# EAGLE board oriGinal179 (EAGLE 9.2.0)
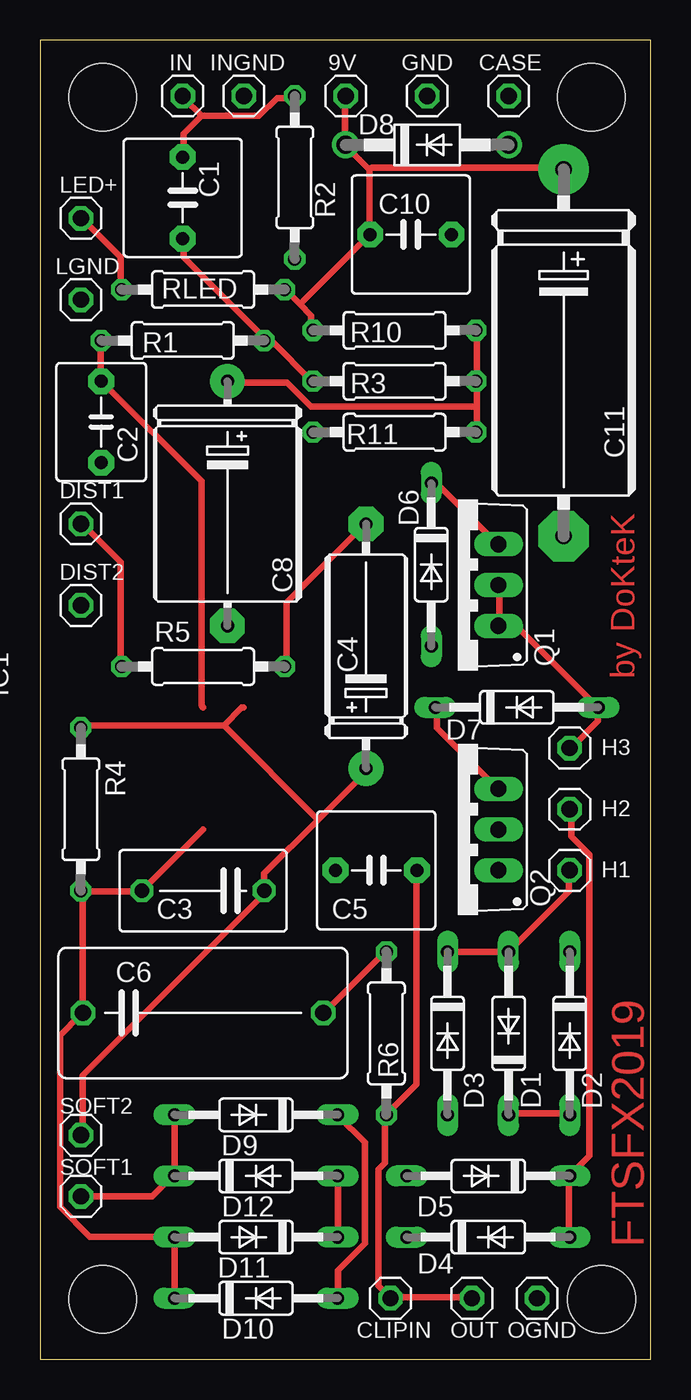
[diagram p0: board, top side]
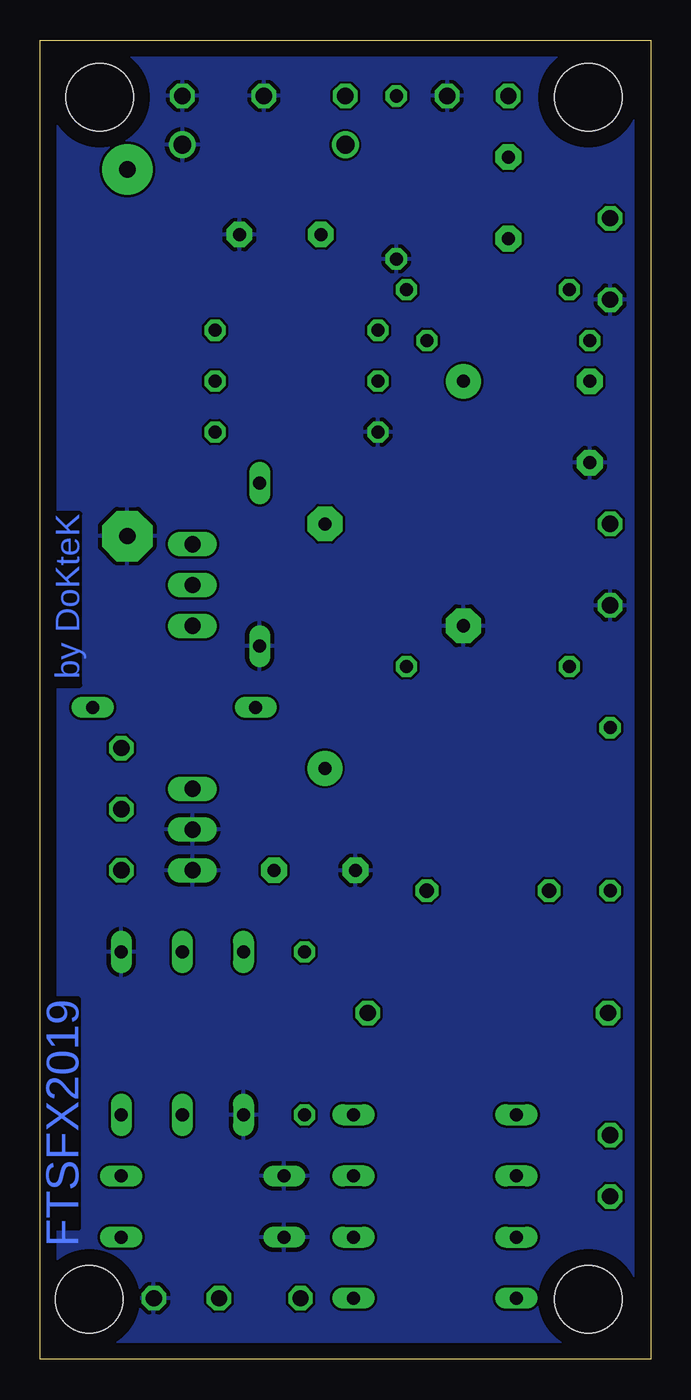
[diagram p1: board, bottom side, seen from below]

Size 38.08 x 82.22 mm. Coordinates in mm from the lower left corner, seen from the top.
Outline: 0,0 38.08,0 38.08,82.22 0,82.22 0,0
Copper layers (1*16): Top 0.035mm / dielectric 1.5mm / Bottom 0.035mm
Design rules "default": minimum track width 6mil, minimum drill 0.35mm, track to track 6mil, track to pad 6mil, pad to pad 6mil, via to via 6mil, smd to smd 6mil, copper to edge 40mil, drill to drill 6mil, minimum pad ring 10mil, minimum via ring 8mil, stop-mask expansion 4mil, vias tented up to drill 0mil, thermal gap 10mil
Net classes: 0 default: width 0.406 mm, drill 0.032 mm; 1 GND: width 24 mm, drill 0.032 mm
Holes 4.2 mm at 3.89,3.74 35.01,3.74 3.89,78.67 34.37,78.67

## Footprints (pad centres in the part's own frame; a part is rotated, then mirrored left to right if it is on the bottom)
1X01 = drill 1.016 octagon: 1 0,0
C5B7.2 = drill 0.813 pad 1.6 octagon: 1 -2.54,0; 2 2.54,0
C5B5.5 = drill 0.813 pad 1.6 octagon: 1 -2.54,0; 2 2.54,0
C075-052X106 = drill 0.914 octagon: 1 -3.81,0; 2 3.81,0
E15-5 = drill 0.813 pad 2.159: + -7.62,0 | drill 0.813 pad 2.159 octagon: - 7.62,0
C150-084X183 = drill 1.016 octagon: 1 -7.493,0; 2 7.493,0
E15-9 = drill 0.813 pad 2.159: + -7.62,0 | drill 0.813 pad 2.159 octagon: - 7.62,0
E22-9 = drill 1.016 pad 3.15: + -11.43,0 | drill 1.016 pad 3.15 octagon: - 11.43,0
DO35-10 = drill 0.813 long: A 5.08,0; C -5.08,0
DO41-10 = drill 1.118: A 5.08,0; C -5.08,0
DIL08 = drill 0.813 pad 1.27: 1 -3.81,-3.81; 2 -1.27,-3.81; 3 1.27,-3.81; 4 3.81,-3.81; 5 3.81,3.81; 6 1.27,3.81; 7 -1.27,3.81; 8 -3.81,3.81
TO220BV = drill 1.016 long: D 0,-2.54; G -2.54,-2.54; S 2.54,-2.54
0207/10 = drill 0.813 octagon: 1 -5.08,0; 2 5.08,0

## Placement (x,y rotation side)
9V  9V  [1X01]  19.05,78.74 0 top
C1  220n  [C5B7.2]  8.89,72.39 270 top
C2  2.2n  [C5B5.5]  3.81,58.42 90 top
C3  3.9n  [C075-052X106]  10.16,29.21 180 top
C4  4.7u  [E15-5]  20.32,44.45 90 top
C5  1n  [C5B7.2]  20.95,30.48 180 top
C6  1u  [C150-084X183]  10.16,21.59 0 top
C8  47u  [E15-9]  11.68,53.34 270 top
C10  100n  [C5B7.2]  23.11,70.1 0 top
C11  100u  [E22-9]  32.64,62.74 270 top
CASE  CASEGND  [1X01]  29.21,78.74 0 top
CLIPIN  CLIPIN  [1X01]  21.84,3.81 0 top
D1  1N4148DO35-10  [DO35-10]  29.21,20.32 90 top
D2  1N4148DO35-10  [DO35-10]  33.02,20.32 270 top
D3  1N4148DO35-10  [DO35-10]  25.4,20.32 270 top
D4  1N4148DO35-10  [DO35-10]  27.94,7.62 0 top
D5  1N4148DO35-10  [DO35-10]  27.94,11.43 180 top
D6  1N4148DO35-10  [DO35-10]  24.38,49.53 270 top
D7  1N4148DO35-10  [DO35-10]  29.72,40.64 0 top
D8  1N4004  [DO41-10]  24.13,75.69 0 top
D9  1N4148DO35-10  [DO35-10]  13.46,15.24 180 top
D10  1N4148DO35-10  [DO35-10]  13.46,3.81 0 top
D11  1N4148DO35-10  [DO35-10]  13.46,7.62 180 top
D12  1N4148DO35-10  [DO35-10]  13.46,11.43 0 top
DIST1  DIST1  [1X01]  2.54,52.07 0 top
DIST2  DIST2  [1X01]  2.54,46.99 0 top
GND  GND  [1X01]  24.13,78.74 0 top
H1  HARD1  [1X01]  33.02,30.48 0 top
H2  HARD2  [1X01]  33.02,34.29 0 top
H3  HARD3  [1X01]  33.02,38.1 0 top
IC1  DIST  [DIL08]  not placed on the board
IN  IN  [1X01]  8.89,78.74 0 top
INGND  INGND  [1X01]  12.7,78.74 0 top
LED+  LED+  [1X01]  2.54,71.12 0 top
LGND  LGND  [1X01]  2.54,66.04 0 top
OGND  OGND  [1X01]  30.99,3.81 0 top
OUT  OUT  [1X01]  26.92,3.81 0 top
Q1  IRF520  [TO220BV]  26.04,48.26 90 top
Q2  IRF520  [TO220BV]  26.04,33.02 90 top
R1  470R  [0207/10]  8.89,63.5 0 top
R2  1M  [0207/10]  15.88,73.66 270 top
R3  47K  [0207/10]  22.1,60.96 180 top
R4  10K  [0207/10]  2.54,34.29 270 top
R5  47R  [0207/10]  10.16,43.18 0 top
R6  10K  [0207/10]  21.59,20.32 90 top
R10  47K  [0207/10]  22.1,64.14 0 top
R11  47K  [0207/10]  22.1,57.78 180 top
RLED  RLED  [0207/10]  10.16,66.67 180 top
SOFT1  SOFT1  [1X01]  2.54,10.16 0 top
SOFT2  SOFT2  [1X01]  2.54,13.97 0 top

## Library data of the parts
9V CASE CLIPIN DIST1 DIST2 GND H1-H3 IN INGND LED+ LGND OGND OUT SOFT1 SOFT2 = pinhead
C1 C2 C5 C10 = capacitor-wima
C3 C4 C6 C8 C11 = rcl; SPICEPREFIX: C
D1-D12 = diode
IC1 = linear
Q1 Q2 = transistor-power
R1-R6 R10 R11 RLED = rcl; SPICEPREFIX: R

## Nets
+4.1V: C8.+ R3.1 R10.2 R11.1
+12V: 9V.1 C10.1 C11.+ D8.C R10.1 RLED.1
GND [GND]: C2.1 C5.2 C8.- C10.2 C11.- CASE.1 D2.C D3.A D4.C D5.A D6.A D8.A DIST2.1 GND.1 INGND.1 LGND.1 OGND.1 Q2.D Q2.G R2.2 R11.2
N$1: C1.1 IN.1 R2.1
N$2: C1.2 R1.2 R3.2
N$3: C2.2 R1.1
N$4: C4.- R5.2
N$5: C3.1 C4.+ R4.1 SOFT2.1
N$6: D9.A D12.C SOFT1.1
N$7: DIST1.1 R5.1
N$8: C5.1 CLIPIN.1 OUT.1 R6.1
N$9: D6.C Q1.S
N$10: D7.A H3.1 Q1.D Q1.G
N$11: D11.C D12.A
N$12: D7.C Q2.S
N$13: D4.A D5.C H2.1
N$14: D9.C D10.A
N$16: D1.C D2.A
N$17: D1.A D3.C H1.1
N$19: C3.2 C6.1 D10.C D11.A R4.2
N$20: LED+.1 RLED.2
N$21: C6.2 R6.2

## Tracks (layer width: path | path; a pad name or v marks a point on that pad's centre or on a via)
+4.1V
  Top 0.406: 27.24,59.39 27.24,60.87 R3.1 27.24,61.15 27.24,64.08 R10.2 | 27.24,59.39 27.24,57.8 R11.1 | 27.24,59.39 16.88,59.39 15.39,60.87 11.73,60.87 C8.+
+12V
  Top 0.406: 16.2,65.76 15.37,66.6 RLED.1 | 16.2,65.76 16.9,65.06 16.9,64.22 R10.1 | 9V.1 19,78.61 19,75.82 D8.C 19.14,75.54 20.54,74.14 | 20.54,74.14 20.54,70.23 C10.1 20.54,70.09 16.2,65.76 | C11.+ 32.55,74.28 20.68,74.28 20.54,74.14
GND
  pour Bottom: 0,82.55 38.1,82.55 38.1,0 0,0
N$1
  Top 0.406: 10.06,77.5 13.64,77.5 14.76,78.61 15.79,78.61 R2.1 | 10.06,77.5 8.94,78.61 IN.1 | 10.06,77.5 8.94,76.38 8.94,74.98 C1.1
N$2
  Top 0.406: R3.2 16.9,61.01 14.53,63.39 13.97,63.39 R1.2 13.97,63.66 8.94,68.69 8.94,69.81 C1.2
N$3
  Top 0.406: R1.1 3.77,63.39 3.77,61.01 C2.2 3.91,60.87 10.06,54.72 10.06,40.75 10.16,40.64
N$4
  Top 0.406: R5.2 15.37,43.27 15.37,47.18 20.26,52.07 C4.-
N$5
  Top 0.406: 11.46,39.5 2.65,39.5 R4.1 | 11.46,39.5 12.57,40.62 12.7,40.64 | 17.32,33.63 20.4,36.7 C4.+ | 17.32,33.63 13.97,30.28 C3.1 13.97,29.02 2.65,17.7 2.65,14.07 SOFT2.1 | 17.32,33.63 11.46,39.5
N$6
  Top 0.406: D9.A D12.C 8.24,11.42 6.99,10.16 SOFT1.1
N$7
  Top 0.406: R5.1 5.03,43.27 5.03,49.69 2.65,52.07 DIST1.1
N$8
  Top 0.406: OUT.1 26.82,3.87 21.93,3.87 CLIPIN.1 21.79,3.87 21.09,4.57 21.09,11.84 21.51,12.25 21.51,15.19 R6.1 21.65,15.33 23.47,17.14 23.47,30.42 C5.1
N$9
  Top 0.406: D6.C 24.45,54.58 24.73,54.58 28.5,50.81 Q1.S
N$10
  Top 0.406: Q1.D 28.64,48.16 28.64,45.78 Q1.G 28.78,45.64 29.76,45.64 34.65,40.75 D7.A 34.78,40.62 34.78,39.78 33.11,38.1 H3.1
N$11
  Top 0.406: D11.C 18.58,7.64 18.58,11.42 D12.A
N$12
  Top 0.406: D7.C 24.73,40.62 24.73,39.36 28.5,35.59 Q2.S
N$13
  Top 0.406: D4.A 32.97,7.64 32.97,11.42 D5.C 33.11,11.56 34.25,12.7 34.25,31.46 33.11,32.6 33.11,34.19 H2.1
N$14
  Top 0.406: D10.A 18.58,3.87 18.58,5.55 20.26,7.23 20.26,13.51 18.58,15.19 D9.C
N$16
  Top 0.406: D1.C 29.34,15.33 32.97,15.33 D2.A
N$17
  Top 0.406: D3.C 25.43,25.39 29.2,25.39 D1.A 32.97,29.16 32.97,30.42 H1.1
N$19
  Top 0.406: D10.C D11.A 8.24,7.64 3.1,7.64 1.25,9.5 1.25,20.21 2.52,21.48 C6.1 2.65,21.62 2.65,29.02 R4.2 2.65,29.16 6.29,29.16 C3.2 6.43,29.3 10.06,32.93 10.16,33.02
N$20
  Top 0.406: RLED.2 5.03,66.74 5.03,68.69 2.65,71.07 LED+.1
N$21
  Top 0.406: R6.2 21.51,25.39 17.74,21.62 C6.2

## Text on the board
Top: by DoKteK | FTSFX2019
Bottom: by DoKteK | FTSFX2019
